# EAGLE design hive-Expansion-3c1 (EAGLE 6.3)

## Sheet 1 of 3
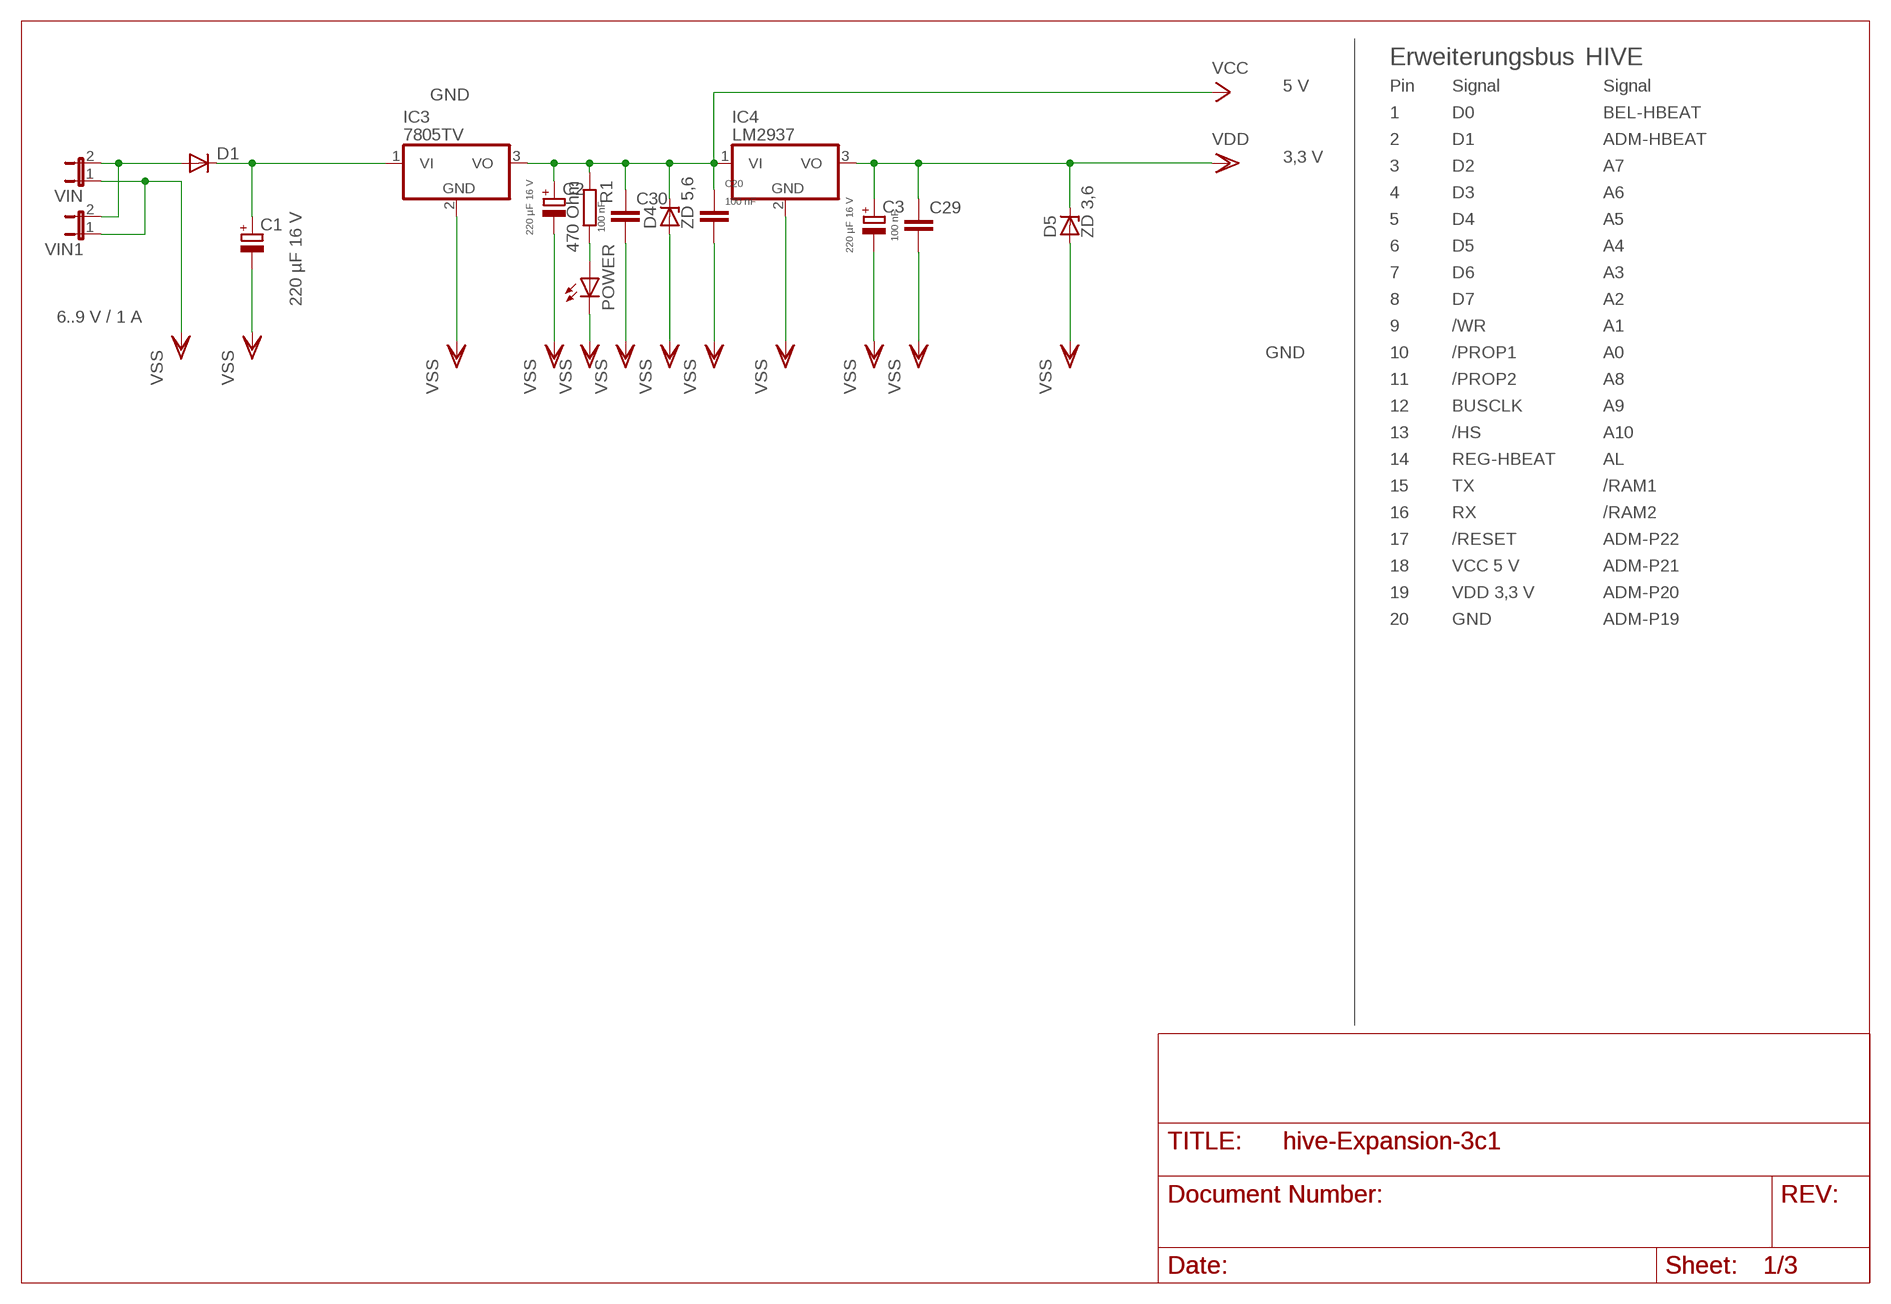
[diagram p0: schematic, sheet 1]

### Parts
C1  220 µF 16 V  CPOL-EUE3.5-10  [E3,5-10]
C2  220 µF 16 V  CPOL-EUE3.5-10  [E3,5-10]
C3  220 µF 16 V  CPOL-EUE3.5-10  [E3,5-10]
C20  100 nF  C5/2.5  [C5B2.5]
C29  100 nF  C5/2.5  [C5B2.5]
C30  100 nF  C5/2.5  [C5B2.5]
D1  DIODE-D-7.5  [D-7.5]
D4  ZD 5,6  ZENER-DIODEDO34-7  [DO34Z7]
D5  ZD 3,6  ZENER-DIODEDO34-7  [DO34Z7]
IC3  7805TV  [TO220V]
IC4  LM2937  7805TV  [TO220V]
POWER  LED5MM  [LED5MM]
R1  470 Ohm  R-EU_0204/2V  [0204V]
VIN  JP1E  [JP1]
VIN1  JP1E  [JP1]

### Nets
N$1 [Power]: D1.A VIN1.2 VIN.2
N$2 [Power]: C1.+ D1.C IC3.1(VI)
N$5: POWER.A R1.2
VCC [Power]: C2.+ C20.1 C30.1 D4.C IC3.3(VO) IC4.1(VI) R1.1 ; also sheet 3
VDD [Power]: C3.+ C29.1 D5.C IC4.3(VO) ; also sheet 2,3
VSS [Power]: C1.- C2.- C3.- C20.2 C29.2 C30.2 D4.A D5.A IC3.2(GND) IC4.2(GND) POWER.K(C) VIN1.1 VIN.1 ; also sheet 2,3

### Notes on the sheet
- Erweiterungsbus | HIVE
- 5 V | Pin | Signal | Signal
- GND
- 1 | D0 | BEL-HBEAT
- 2 | D1 | ADM-HBEAT
- 3,3 V
- 3 | D2 | A7
- 4 | D3 | A6
- 5 | D4 | A5
- 6 | D5 | A4
- 7 | D6 | A3
- 8 | D7 | A2
- 6..9 V / 1 A
- 9 | /WR | A1
- GND | 10 | /PROP1 | A0
- 11 | /PROP2 | A8
- 12 | BUSCLK | A9
- 13 | /HS | A10
- 14 | REG-HBEAT | AL
- 15 | TX | /RAM1
- 16 | RX | /RAM2
- 17 | /RESET | ADM-P22
- 18 | VCC 5 V | ADM-P21
- 19 | VDD 3,3 V | ADM-P20
- 20 | GND | ADM-P19

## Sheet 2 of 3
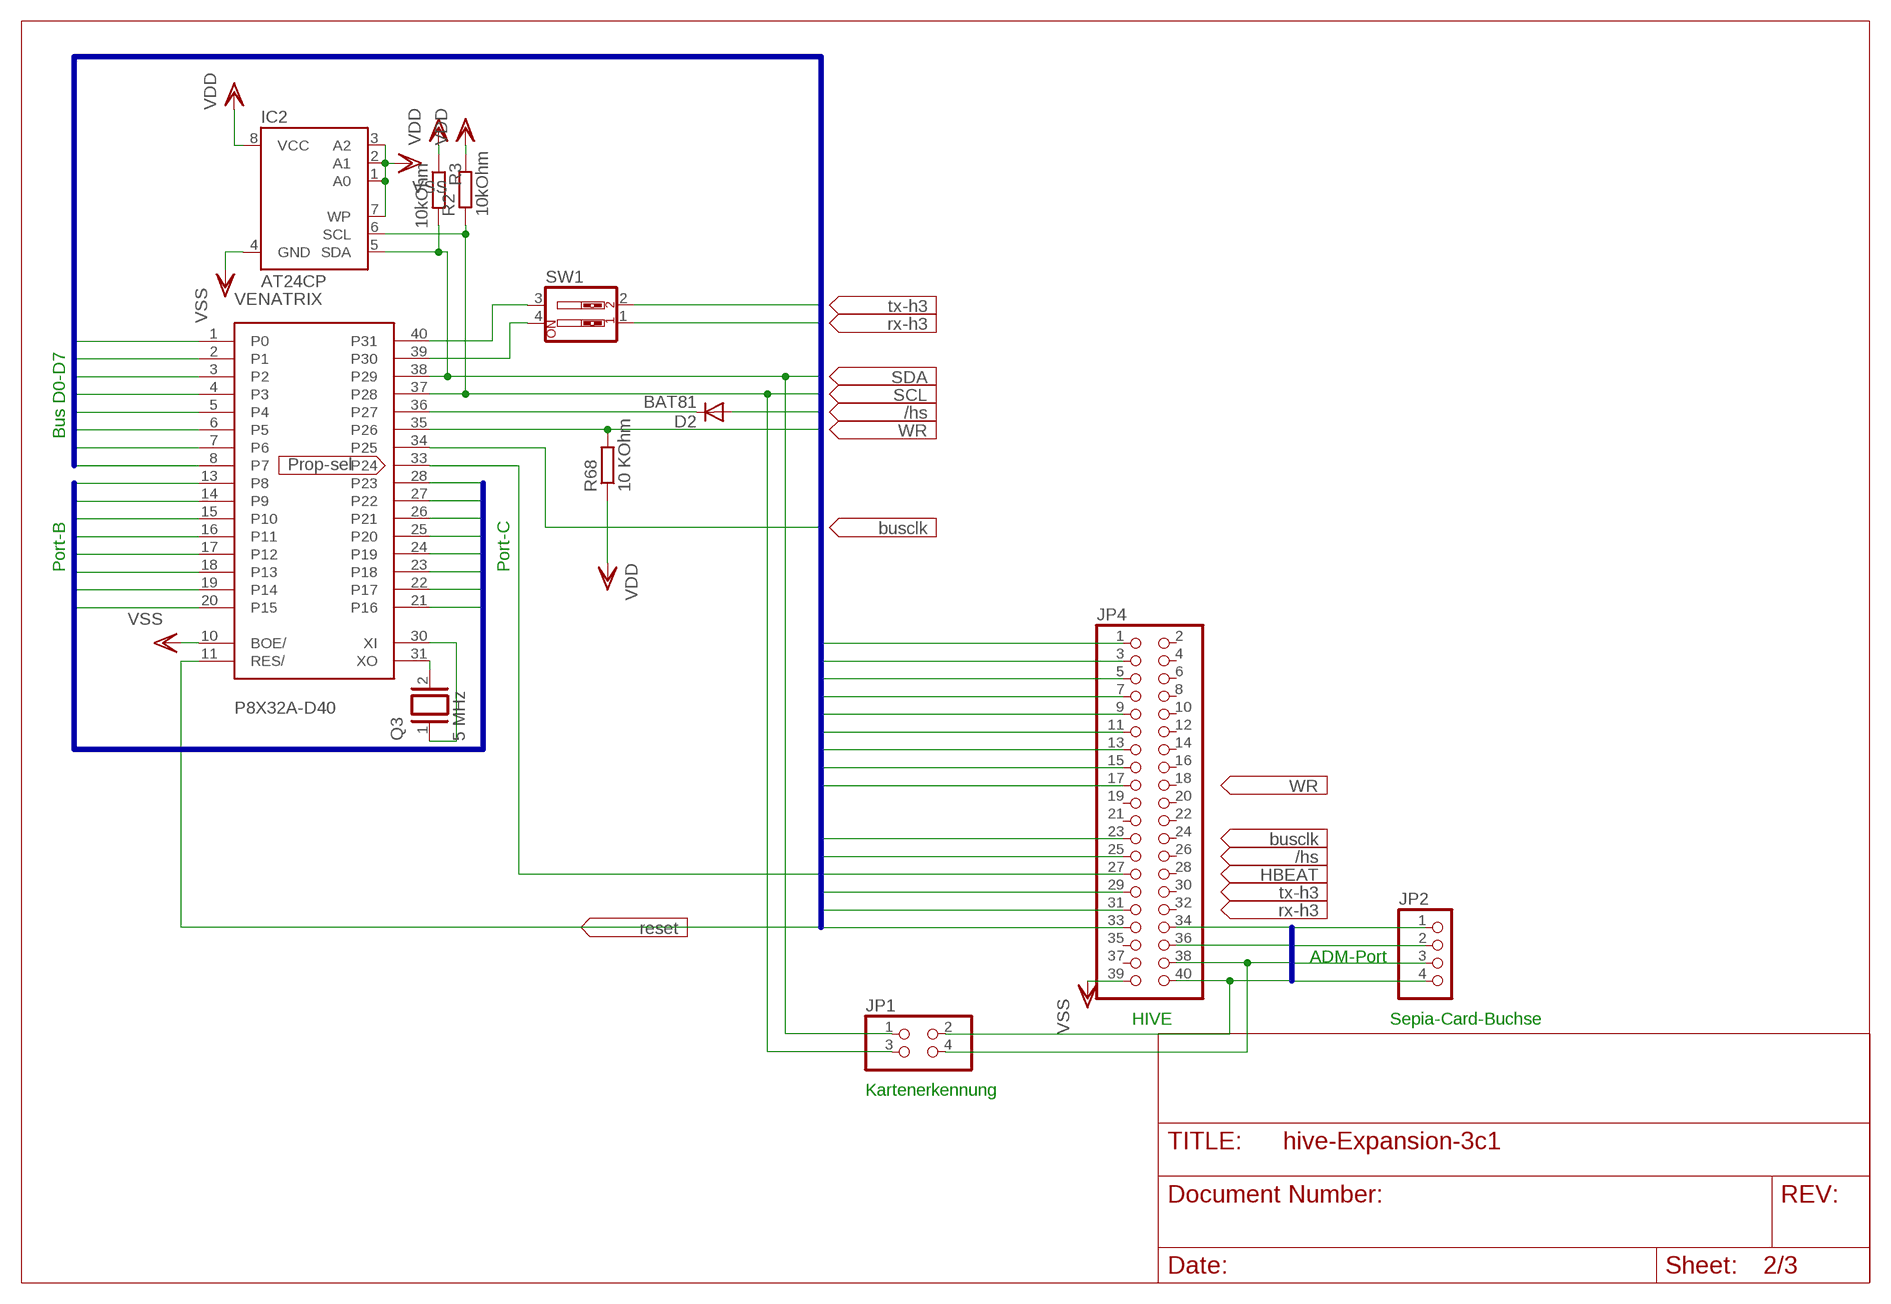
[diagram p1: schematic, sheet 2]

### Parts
D2  BAT81  [DO34-7]
IC2  AT24CP  [DIL08]
JP1  PINHD-2X2  [2X02]
JP2  PINHD-1X4  [1X04]
JP4  PINHD-2X20  [2X20]
Q3  5 MHz  XTAL/S  [QS]
R2  10kOhm  R-EU_0204/2V  [0204V]
R3  10kOhm  R-EU_0204/2V  [0204V]
R68  10 KOhm  R-EU_0204/2V  [0204V]
SW1  SW_DIP-2  [EDG-02]
VENATRIX  P8X32A-D40  [P8X32A-D40]

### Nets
EXPANSIONA1: JP4.1 VENATRIX.1(P0) ; also sheet 3
EXPANSIONA2: JP4.3 VENATRIX.2(P1) ; also sheet 3
EXPANSIONA3: JP4.5 VENATRIX.3(P2) ; also sheet 3
EXPANSIONA4: JP4.7 VENATRIX.4(P3) ; also sheet 3
EXPANSIONA5: JP4.9 VENATRIX.5(P4) ; also sheet 3
EXPANSIONA6: JP4.11 VENATRIX.6(P5) ; also sheet 3
EXPANSIONA7: JP4.13 VENATRIX.7(P6) ; also sheet 3
EXPANSIONA8: JP4.15 VENATRIX.8(P7) ; also sheet 3
EXPANSIONA9: JP4.17 R68.2 VENATRIX.35(P26) ; also sheet 3
EXPANSIONA10: IC2.5(SDA) JP1.1 R3.2 VENATRIX.38(P29) ; also sheet 3
EXPANSIONA11: IC2.6(SCL) JP1.3 R2.1 VENATRIX.37(P28) ; also sheet 3
EXPANSIONA12: JP4.23 VENATRIX.34(P25) ; also sheet 3
EXPANSIONA13: D2.A JP4.25 ; also sheet 3
EXPANSIONA14: JP4.29 SW1.1 ; also sheet 3
EXPANSIONA15: JP4.31 SW1.2 ; also sheet 3
EXPANSIONA16: JP4.33 VENATRIX.11(RES/) ; also sheet 3
EXPANSIONB1: VENATRIX.13(P8) ; also sheet 3
EXPANSIONB2: VENATRIX.14(P9) ; also sheet 3
EXPANSIONB3: VENATRIX.15(P10) ; also sheet 3
EXPANSIONB4: VENATRIX.16(P11) ; also sheet 3
EXPANSIONB5: VENATRIX.17(P12) ; also sheet 3
EXPANSIONB6: VENATRIX.18(P13) ; also sheet 3
EXPANSIONB7: VENATRIX.19(P14) ; also sheet 3
EXPANSIONB8: VENATRIX.20(P15) ; also sheet 3
EXPANSIONB9: VENATRIX.28(P23) ; also sheet 3
EXPANSIONB10: VENATRIX.27(P22) ; also sheet 3
EXPANSIONB11: VENATRIX.26(P21) ; also sheet 3
EXPANSIONB12: VENATRIX.25(P20) ; also sheet 3
EXPANSIONB13: VENATRIX.24(P19) ; also sheet 3
EXPANSIONB14: VENATRIX.23(P18) ; also sheet 3
EXPANSIONB15: VENATRIX.22(P17) ; also sheet 3
EXPANSIONB16: VENATRIX.21(P16) ; also sheet 3
EXPANSIONB17: JP2.1 JP4.34 ; also sheet 3
EXPANSIONB18: JP2.2 JP4.36 ; also sheet 3
EXPANSIONB19: JP1.4 JP2.3 JP4.38 ; also sheet 3
EXPANSIONB20: JP1.2 JP2.4 JP4.40 ; also sheet 3
N$3: D2.C VENATRIX.36(P27)
N$4: SW1.4 VENATRIX.39(P30)
N$6: SW1.3 VENATRIX.40(P31)
N$7: JP4.27 VENATRIX.33(P24)
N$65: Q3.2 VENATRIX.31(XO)
N$66: Q3.1 VENATRIX.30(XI)
VDD [Power]: IC2.8(VCC) R2.2 R3.1 R68.1 ; also sheet 1,3
VSS [Power]: IC2.1(A0) IC2.2(A1) IC2.3(A2) IC2.4(GND) IC2.7(WP) JP4.39 VENATRIX.10(BOE/) ; also sheet 1,3
Unconnected: JP4.2 JP4.4 JP4.6 JP4.8 JP4.10 JP4.12 JP4.14 JP4.16 JP4.18 JP4.19 JP4.20 JP4.21 JP4.22 JP4.24 JP4.26 JP4.28 JP4.30 JP4.32 JP4.35 JP4.37

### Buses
EXPANSIONA[1..22]
EXPANSIONB[1..22]

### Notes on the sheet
- Bus D0-D7
- Port-B | Port-C
- ADM-Port
- HIVE | Sepia-Card-Buchse
- Kartenerkennung

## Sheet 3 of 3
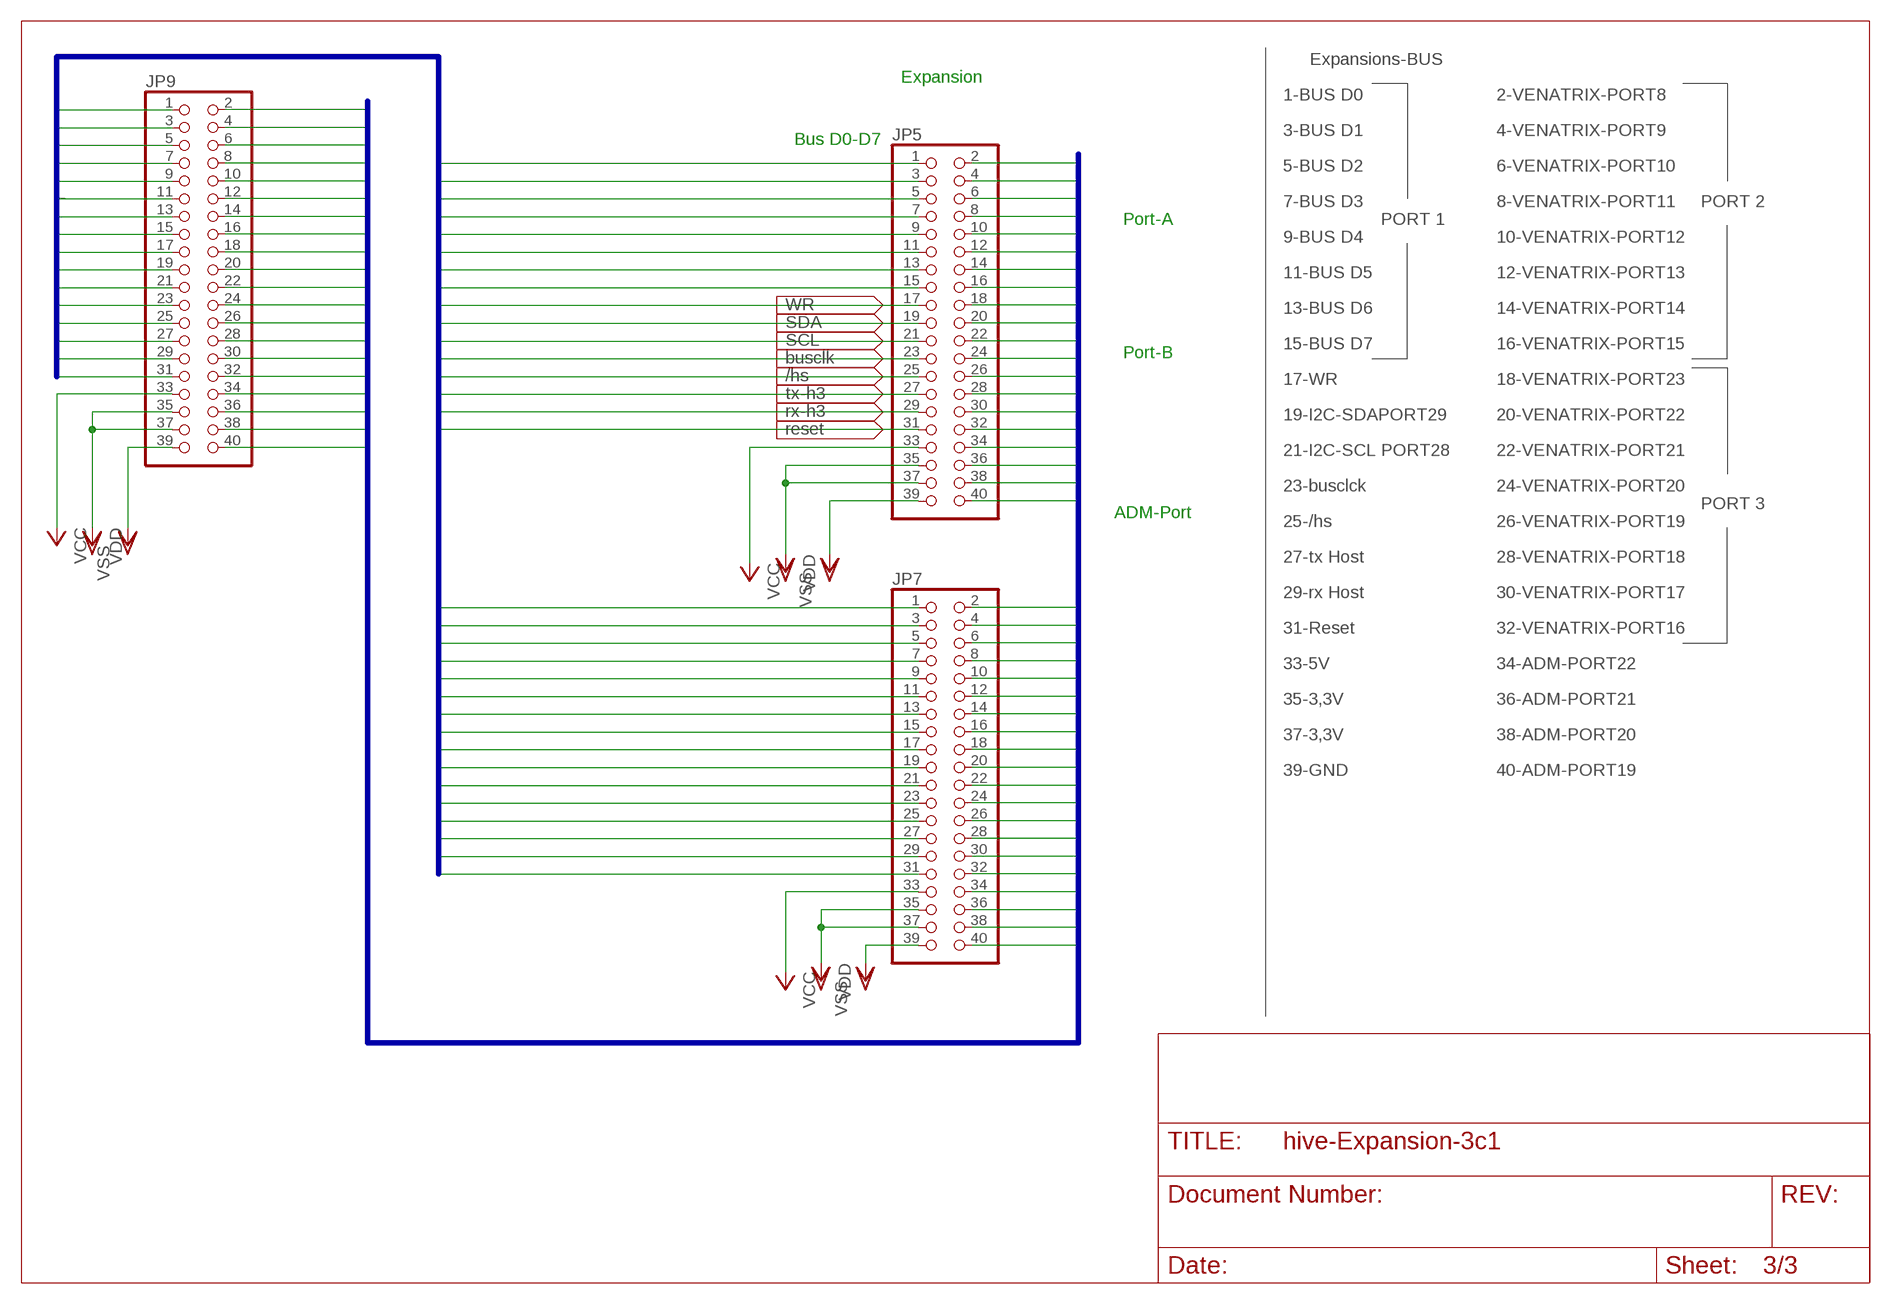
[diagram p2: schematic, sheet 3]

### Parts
JP5  PINHD-2X20  [2X20]
JP7  PINHD-2X20  [2X20]
JP9  PINHD-2X20  [2X20]

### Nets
EXPANSIONA1: JP5.1 JP7.1 JP9.1 ; also sheet 2
EXPANSIONA2: JP5.3 JP7.3 JP9.3 ; also sheet 2
EXPANSIONA3: JP5.5 JP7.5 JP9.5 ; also sheet 2
EXPANSIONA4: JP5.7 JP7.7 JP9.7 ; also sheet 2
EXPANSIONA5: JP5.9 JP7.9 JP9.9 ; also sheet 2
EXPANSIONA6: JP5.11 JP7.11 JP9.11 ; also sheet 2
EXPANSIONA7: JP5.13 JP7.13 JP9.13 ; also sheet 2
EXPANSIONA8: JP5.15 JP7.15 JP9.15 ; also sheet 2
EXPANSIONA9: JP5.17 JP7.17 JP9.17 ; also sheet 2
EXPANSIONA10: JP5.19 JP7.19 JP9.19 ; also sheet 2
EXPANSIONA11: JP5.21 JP7.21 JP9.21 ; also sheet 2
EXPANSIONA12: JP5.23 JP7.23 JP9.23 ; also sheet 2
EXPANSIONA13: JP5.25 JP7.25 JP9.25 ; also sheet 2
EXPANSIONA14: JP5.27 JP7.27 JP9.27 ; also sheet 2
EXPANSIONA15: JP5.29 JP7.29 JP9.29 ; also sheet 2
EXPANSIONA16: JP5.31 JP7.31 JP9.31 ; also sheet 2
EXPANSIONB1: JP5.2 JP7.2 JP9.2 ; also sheet 2
EXPANSIONB2: JP5.4 JP7.4 JP9.4 ; also sheet 2
EXPANSIONB3: JP5.6 JP7.6 JP9.6 ; also sheet 2
EXPANSIONB4: JP5.8 JP7.8 JP9.8 ; also sheet 2
EXPANSIONB5: JP5.10 JP7.10 JP9.10 ; also sheet 2
EXPANSIONB6: JP5.12 JP7.12 JP9.12 ; also sheet 2
EXPANSIONB7: JP5.14 JP7.14 JP9.14 ; also sheet 2
EXPANSIONB8: JP5.16 JP7.16 JP9.16 ; also sheet 2
EXPANSIONB9: JP5.18 JP7.18 JP9.18 ; also sheet 2
EXPANSIONB10: JP5.20 JP7.20 JP9.20 ; also sheet 2
EXPANSIONB11: JP5.22 JP7.22 JP9.22 ; also sheet 2
EXPANSIONB12: JP5.24 JP7.24 JP9.24 ; also sheet 2
EXPANSIONB13: JP5.26 JP7.26 JP9.26 ; also sheet 2
EXPANSIONB14: JP5.28 JP7.28 JP9.28 ; also sheet 2
EXPANSIONB15: JP5.30 JP7.30 JP9.30 ; also sheet 2
EXPANSIONB16: JP5.32 JP7.32 JP9.32 ; also sheet 2
EXPANSIONB17: JP5.34 JP7.34 JP9.34 ; also sheet 2
EXPANSIONB18: JP5.36 JP7.36 JP9.36 ; also sheet 2
EXPANSIONB19: JP5.38 JP7.38 JP9.38 ; also sheet 2
EXPANSIONB20: JP5.40 JP7.40 JP9.40 ; also sheet 2
VCC [Power]: JP5.33 JP7.33 JP9.33 ; also sheet 1
VDD [Power]: JP5.35 JP5.37 JP7.35 JP7.37 JP9.35 JP9.37 ; also sheet 1,2
VSS [Power]: JP5.39 JP7.39 JP9.39 ; also sheet 1,2

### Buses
EXPANSIONA[1..22]
EXPANSIONB[1..22]

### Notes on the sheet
- Expansions-BUS
- Expansion
- 1-BUS D0 | 2-VENATRIX-PORT8
- 3-BUS D1 | 4-VENATRIX-PORT9
- Bus D0-D7
- 5-BUS D2 | 6-VENATRIX-PORT10
- 7-BUS D3 | 8-VENATRIX-PORT11 | PORT 2
- Port-A | PORT 1
- 9-BUS D4 | 10-VENATRIX-PORT12
- 11-BUS D5 | 12-VENATRIX-PORT13
- 13-BUS D6 | 14-VENATRIX-PORT14
- 15-BUS D7 | 16-VENATRIX-PORT15
- Port-B
- 17-WR | 18-VENATRIX-PORT23
- 19-I2C-SDAPORT29 | 20-VENATRIX-PORT22
- 21-I2C-SCL PORT28 | 22-VENATRIX-PORT21
- 23-busclck | 24-VENATRIX-PORT20
- PORT 3
- ADM-Port
- 25-/hs | 26-VENATRIX-PORT19
- 27-tx Host | 28-VENATRIX-PORT18
- 29-rx Host | 30-VENATRIX-PORT17
- 31-Reset | 32-VENATRIX-PORT16
- 33-5V | 34-ADM-PORT22
- 35-3,3V | 36-ADM-PORT21
- 37-3,3V | 38-ADM-PORT20
- 39-GND | 40-ADM-PORT19

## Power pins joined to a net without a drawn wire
VDD: VENATRIX.12(VDD) VENATRIX.32(VDD)
VSS: VENATRIX.9(VSS) VENATRIX.29(VSS)

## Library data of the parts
C1-C3 = rcl:CPOL-EU: POLARIZED CAPACITOR, European symbol
C20 C29 C30 = capacitor-wima:C: CAPACITOR
D1 = diode:DIODE-: DIODE
D2 = diode:BAT81: DIODE
D4 D5 = diode:ZENER-DIODE: Z-Diode
IC2 = atmel:AT24C*: 2-wire serial EEPROM; MPN: AT24C1024BW-SH-B; OC_FARNELL: 1362646; OC_NEWARK: 03P2044
IC3 IC4 = linear:78*: Positive VOLTAGE REGULATOR Source: http://cache.national.com/ds/LM/LM78L05.pdf http://www.fairchildsemi.com/ds/LM/LM7805.pdf
JP1 = pinhead:PINHD-2X2: PIN HEADER
JP2 = pinhead:PINHD-1X4: PIN HEADER
JP4 JP5 JP7 JP9 = pinhead:PINHD-2X20: PIN HEADER
POWER = led:LED: LED
Q3 = special:XTAL/S: CRYSTAL
R1-R3 R68 = rcl:R-EU_: RESISTOR, European symbol
SW1 = special:SW_DIP-2: DIP SWITCH
VENATRIX = parallax_propeller:P8X32A-D40
VIN VIN1 = jumper:JP1E: JUMPER

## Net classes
0 default: width 0.254 mm, clearance 0.254 mm
1 Power: width 0.635 mm, drill 0.61 mm, clearance 0.381 mm
2 AudioVideo: width 0.254 mm, clearance 0.254 mm
3 Priority: width 0.279 mm, clearance 0.279 mm

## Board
Hive-Expansionsport-Platine Diese Variante soll Huckepack auf die Hive-Platine montiert werden
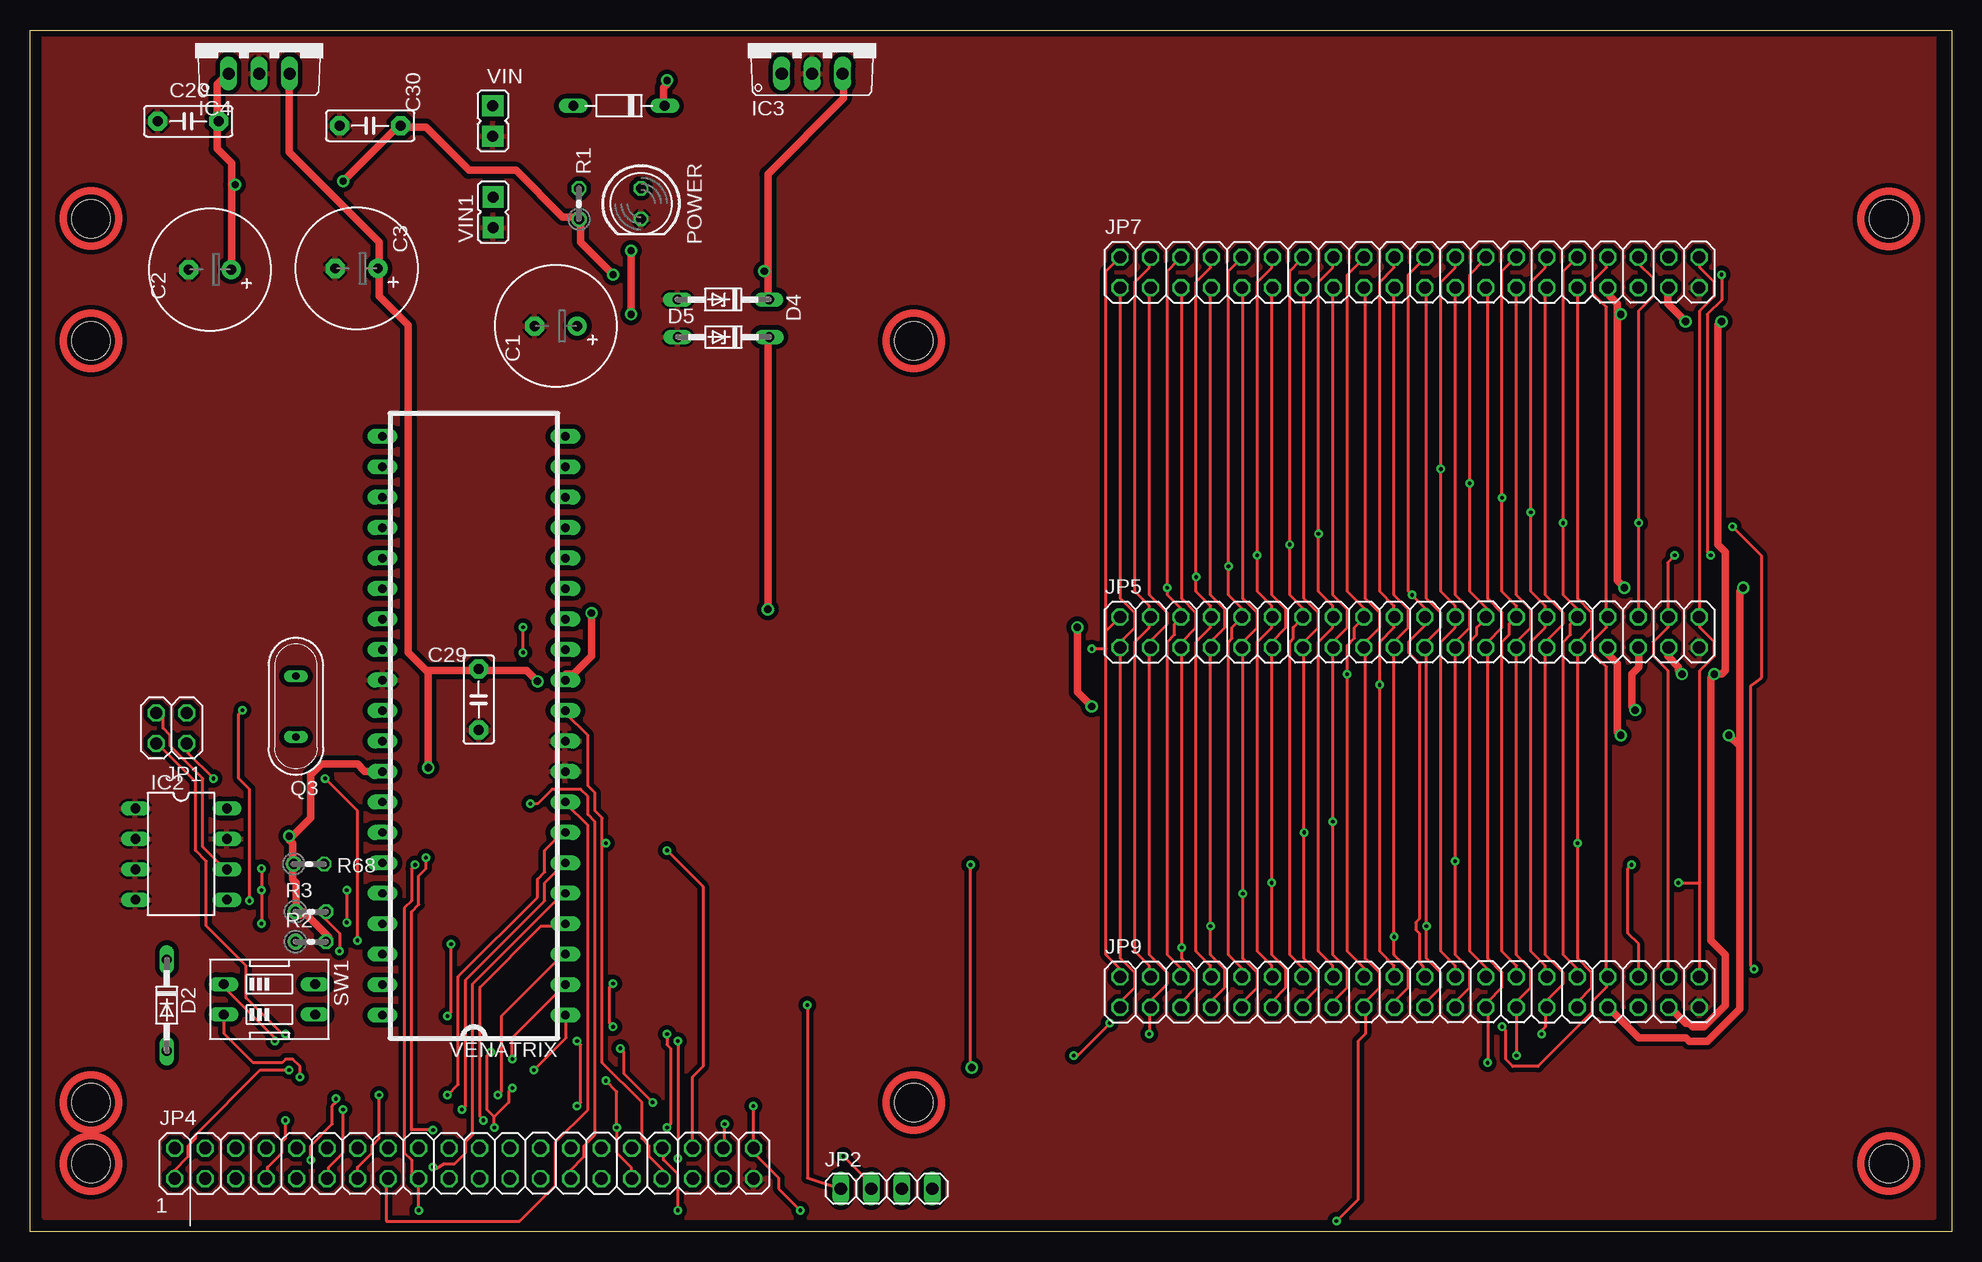
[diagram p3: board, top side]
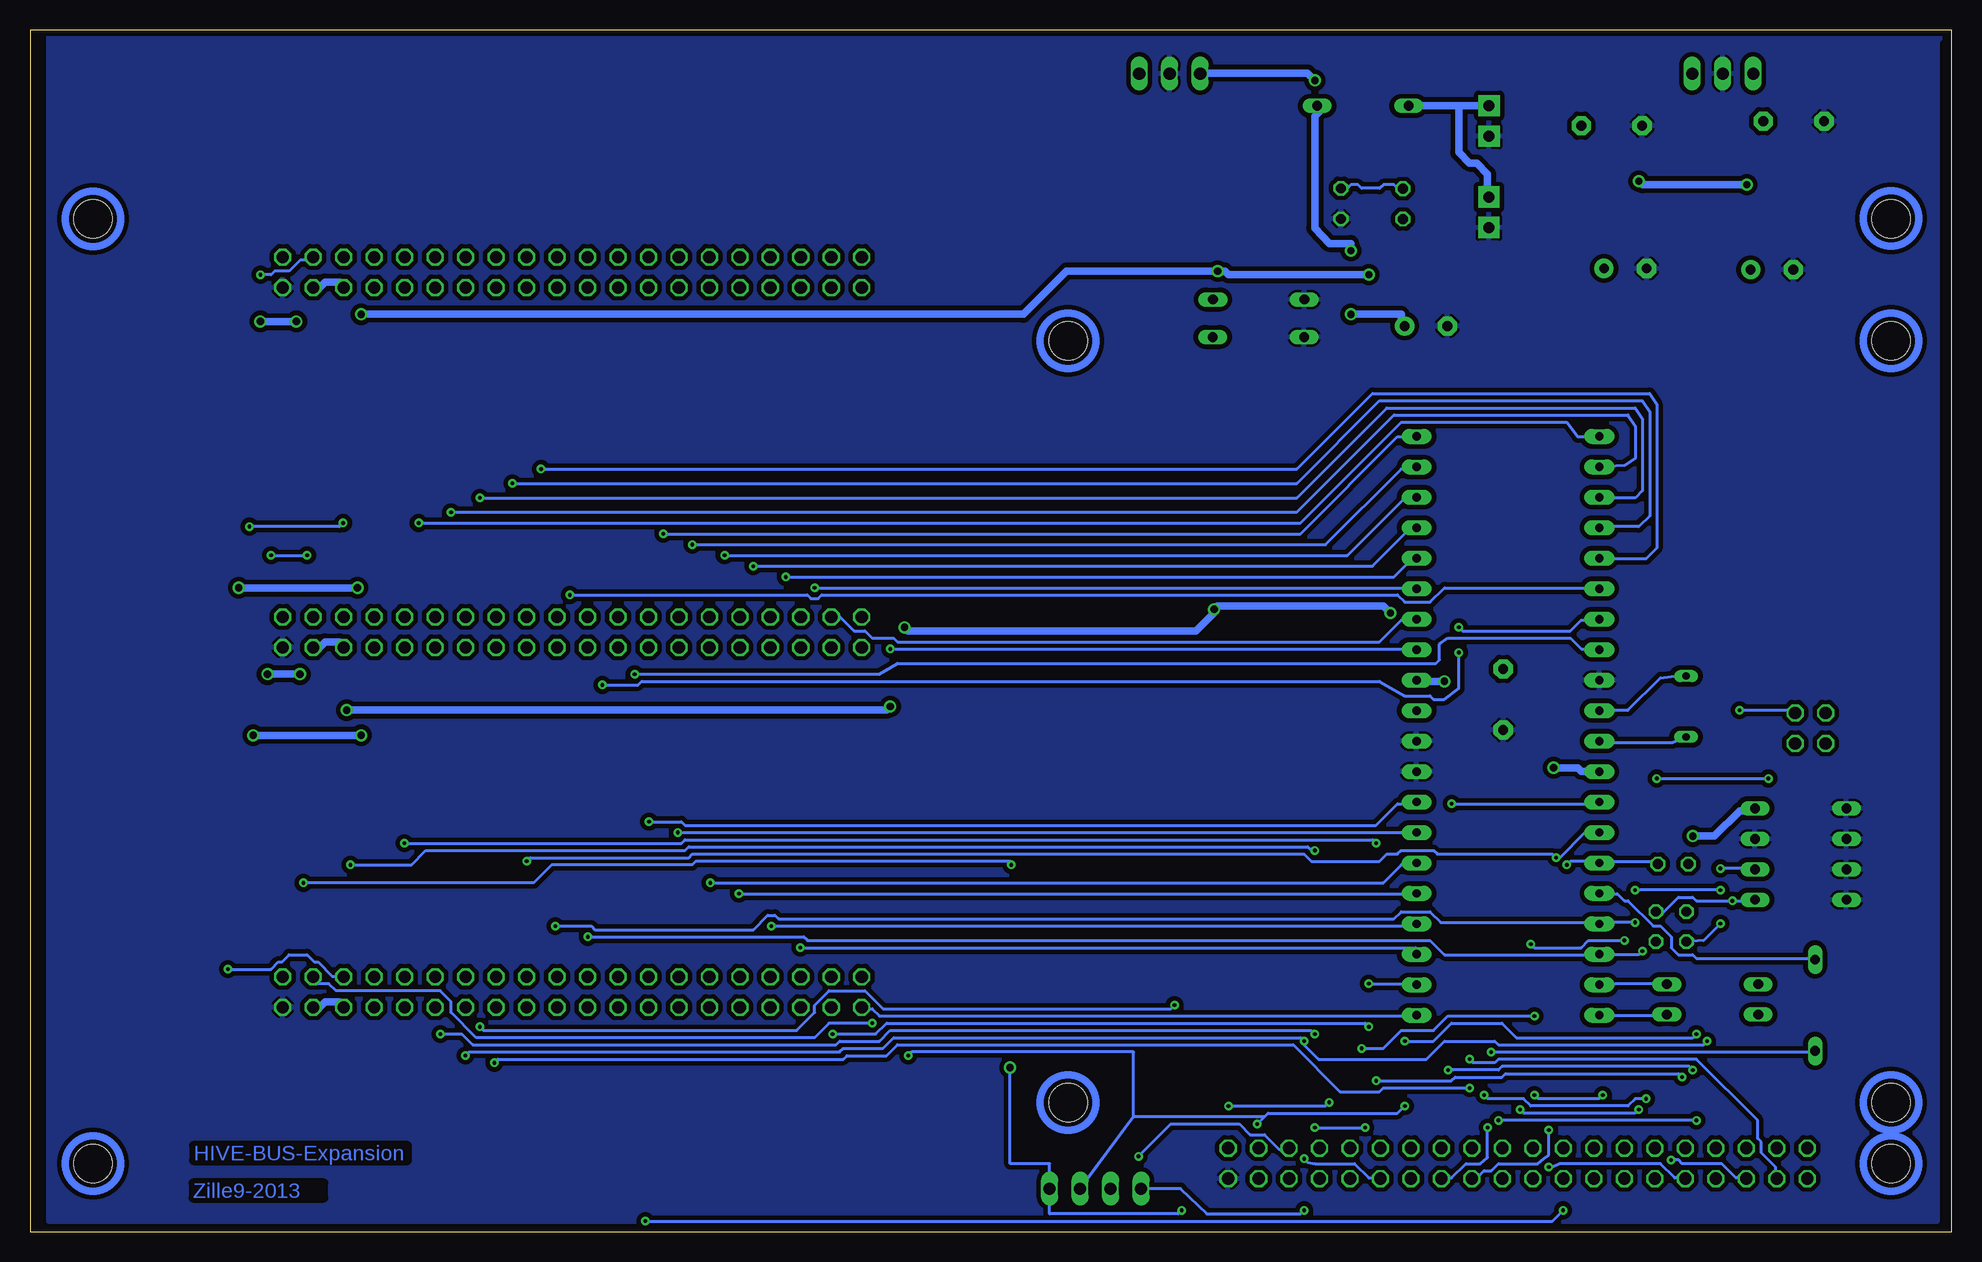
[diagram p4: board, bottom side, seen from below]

Size 160.2 x 100.2 mm. Coordinates in mm from the lower left corner, seen from the top.
Outline: 0,0 0,100.2 160.2,100.2 160.2,0 0,0
Copper layers (1*16): Top 0.035mm / dielectric 1.5mm / Bottom 0.035mm
Design rules "PCB-POOL": minimum track width 6mil, minimum drill 12mil, track to track 6mil, track to pad 6mil, pad to pad 6mil, via to via 6mil, smd to smd 6mil, copper to edge 20mil, drill to drill 8mil, minimum pad ring 8mil, minimum via ring 8mil, stop-mask expansion 3mil, vias tented up to drill 24mil, thermal gap 8mil
Holes 3.2 mm at 73.66,74.3 5.08,74.3 5.08,10.79 73.66,10.79 154.94,84.46 154.94,5.71 5.08,84.45 5.08,5.71

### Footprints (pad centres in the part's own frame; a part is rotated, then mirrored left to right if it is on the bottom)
E3,5-10 = drill 0.813 pad 1.6: + -1.778,0 | drill 0.813 pad 1.6 octagon: - 1.778,0
C5B2.5 = drill 0.813 pad 1.6 octagon: 1 -2.54,0; 2 2.54,0
D-7.5 = drill 0.813 long: A 3.81,0; C -3.81,0
DO34-7 = drill 0.813 long: A 3.81,0; C -3.81,0
DO34Z7 = drill 0.813 long: A 3.81,0; C -3.81,0
DIL08 = drill 0.813 long: 1 -3.81,-3.81; 2 -1.27,-3.81; 3 1.27,-3.81; 4 3.81,-3.81; 5 3.81,3.81; 6 1.27,3.81; 7 -1.27,3.81; 8 -3.81,3.81
TO220V = drill 1.016 long: 1 -2.54,-2.54; 2 0,-2.54; 3 2.54,-2.54
2X02 = drill 1.016 octagon: 1 -1.27,-1.27; 2 -1.27,1.27; 3 1.27,-1.27; 4 1.27,1.27
1X04 = drill 1.016 long: 1 -3.81,0; 2 -1.27,0; 3 1.27,0; 4 3.81,0
2X20 = drill 1.016 octagon: 1 -24.13,-1.27; 2 -24.13,1.27; 3 -21.59,-1.27; 4 -21.59,1.27; 5 -19.05,-1.27; 6 -19.05,1.27; 7 -16.51,-1.27; 8 -16.51,1.27; 9 -13.97,-1.27; 10 -13.97,1.27; 11 -11.43,-1.27; 12 -11.43,1.27; 13 -8.89,-1.27; 14 -8.89,1.27; 15 -6.35,-1.27; 16 -6.35,1.27; 17 -3.81,-1.27; 18 -3.81,1.27; 19 -1.27,-1.27; 20 -1.27,1.27; 21 1.27,-1.27; 22 1.27,1.27; 23 3.81,-1.27; 24 3.81,1.27; 25 6.35,-1.27; 26 6.35,1.27; 27 8.89,-1.27; 28 8.89,1.27; 29 11.43,-1.27; 30 11.43,1.27; 31 13.97,-1.27; 32 13.97,1.27; 33 16.51,-1.27; 34 16.51,1.27; 35 19.05,-1.27; 36 19.05,1.27; 37 21.59,-1.27; 38 21.59,1.27; 39 24.13,-1.27; 40 24.13,1.27
LED5MM = drill 0.813 octagon: A -1.27,0; K 1.27,0
QS = drill 0.61 long: 1 -2.54,0; 2 2.54,0
0204V = drill 0.813 octagon: 1 -1.27,0; 2 1.27,0
EDG-02 = drill 0.813 long: 1 -1.27,-3.81; 2 1.27,-3.81; 3 1.27,3.81; 4 -1.27,3.81
P8X32A-D40 = drill 0.7 pad 1.27 long: 1 -7.62,23.495; 2 -7.62,20.955; 3 -7.62,18.415; 4 -7.62,15.875; 5 -7.62,13.335; 6 -7.62,10.795; 7 -7.62,8.255; 8 -7.62,5.715; 9 -7.62,3.175; 10 -7.62,0.635; 11 -7.62,-1.905; 12 -7.62,-4.445; 13 -7.62,-6.985; 14 -7.62,-9.525; 15 -7.62,-12.065; 16 -7.62,-14.605; 17 -7.62,-17.145; 18 -7.62,-19.685; 19 -7.62,-22.225; 20 -7.62,-24.765; 21 7.62,-24.765; 22 7.62,-22.225; 23 7.62,-19.685; 24 7.62,-17.145; 25 7.62,-14.605; 26 7.62,-12.065; 27 7.62,-9.525; 28 7.62,-6.985; 29 7.62,-4.445; 30 7.62,-1.905; 31 7.62,0.635; 32 7.62,3.175; 33 7.62,5.715; 34 7.62,8.255; 35 7.62,10.795; 36 7.62,13.335; 37 7.62,15.875; 38 7.62,18.415; 39 7.62,20.955; 40 7.62,23.495
JP1 = drill 0.914 pad 1.778 square: 1 0,-1.27; 2 0,1.27

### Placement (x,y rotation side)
C1  43.84,75.52 180 top
C2  15,80.22 180 top
C3  27.22,80.32 180 top
C20  13.19,92.59 180 top
C29  37.4,44.39 270 top
C30  28.36,92.22 180 top
D1  49.09,93.89 180 top
D2  11.4,18.9 270 top
D4  57.79,77.73 180 top
D5  57.81,74.6 180 top
IC2  12.6,31.5 270 top
IC3  65.2,99.1 0 top
IC4  19.1,99.1 0 top
JP1  11.8,42 180 top
JP2  71.4,3.6 0 top
JP4  36.2,5.71 0 top
JP5  115,50 0 top
JP7  115,80 0 top
JP9  115,20 0 top
POWER  50.93,85.73 270 top
Q3  22.16,43.8 270 top
R1  45.76,85.71 90 top
R2  23.4,24.2 0 top
R3  23.4,26.7 0 top
R68  23.24,30.67 0 top
SW1  19.95,19.39 270 top
VENATRIX  37,41.56 180 top
VIN  38.58,92.62 0 top
VIN1  38.6,85 0 top

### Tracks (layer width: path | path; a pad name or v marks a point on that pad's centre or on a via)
EXPANSIONA1  (via drill 0.3)
  Top 0.254: v42,13.5 44.7,16.2 44.7,18 VENATRIX.1 | v21.6,13.5 19.2,13.5 13.8,8.1 13.8,7.8 13.2,7.2 13.2,6.3 12,5.1 12,4.5 JP4.1 | JP9.1 90.9,18.9 90.9,19.2 92.1,20.4 92.1,21.6 90.9,22.8 90.9,48.6 JP5.1 90.9,48.9 90.9,49.2 92.1,50.4 92.1,51.6 90.9,52.8 90.9,78.6 JP7.1
  Bottom 0.254: v42,13.5 37.8,13.5 37.5,13.8 21.9,13.8 v21.6,13.5 | VENATRIX.1 44.7,18 89.4,18 90,18.6 90.6,18.6 JP9.1
EXPANSIONA2  (via drill 0.3)
  Top 0.254: v40.2,14.4 40.2,16.2 44.4,20.4 VENATRIX.2 | JP7.3 93.3,78.6 93.3,53.1 94.8,51.6 94.8,50.7 93.3,49.2 93.3,48.9 JP5.3 93.3,48.6 93.3,23.1 94.8,21.6 94.8,20.7 93.3,19.2 93.3,18.9 JP9.3 93.3,18.6 v93.3,16.5 | v48.6,20.7 48.3,20.4 48.3,17.4 v48.6,17.1
  Bottom 0.254: v40.2,14.4 39.9,14.1 38.1,14.1 37.8,14.4 21.3,14.4 16.2,9.3 16.2,7.8 15.9,7.5 15.9,6.6 14.7,5.4 14.7,4.5 JP4.3 | v48.6,20.7 44.7,20.7 VENATRIX.2 | v48.6,17.1 48.9,17.4 88.8,17.4 89.7,16.5 v93.3,16.5
EXPANSIONA3  (via drill 0.3)
  Top 0.254: v39,11.4 39.3,11.7 39.3,18 44.4,23.1 VENATRIX.3 | v25.5,11.1 25.5,10.8 25.2,10.5 25.2,9 23.4,7.2 v23.4,6 | JP9.5 96,18.9 96,19.2 97.2,20.4 97.2,21.6 96,22.8 v96,23.7 96,48.6 JP5.5 96,48.9 96,49.2 97.2,50.4 97.2,51.6 96,52.8 96,78.6 JP7.5
  Bottom 0.254: v39,11.4 38.7,11.1 35.7,11.1 35.1,10.5 27,10.5 26.4,11.1 v25.5,11.1 | v23.4,6 22.8,6 22.5,5.7 19.2,5.7 18,4.5 17.4,4.5 JP4.5 | v96,23.7 44.7,23.7 VENATRIX.3
EXPANSIONA4  (via drill 0.3)
  Top 0.254: v37.8,9.3 37.5,9.6 37.5,20.4 42.6,25.5 44.4,25.5 VENATRIX.4 | v21.3,9.3 21.3,7.8 21,7.5 21,6.6 19.8,5.4 19.8,4.5 JP4.7 | JP9.7 98.4,18.9 98.4,19.2 99.6,20.4 99.6,21.9 98.4,23.1 v98.4,25.5 98.4,48.6 JP5.7 98.4,48.9 98.4,49.2 99.6,50.4 99.6,51.9 98.4,53.1 98.4,78.6 JP7.7
  Bottom 0.254: v21.3,9.3 v37.8,9.3 | v98.4,25.5 44.7,25.5 VENATRIX.4
EXPANSIONA5  (via drill 0.3)
  Top 0.254: v33.6,5.4 33.9,5.3 34.5,5.7 35.4,5.7 36.3,6.6 36.3,7.5 36.9,8.1 36.9,20.7 44.4,28.2 VENATRIX.5 | JP9.9 101.1,18.9 101.1,19.2 102.3,20.4 102.3,21.6 101.1,22.8 v101.1,28.2 101.1,48.6 JP5.9 101.1,48.9 101.1,49.2 102.3,50.4 102.3,51.6 101.1,52.8 101.1,78.6 JP7.9
  Bottom 0.254: v33.6,5.4 33.3,5.4 32.7,5.7 24.3,5.7 23.1,4.5 22.5,4.5 JP4.9 | v101.1,28.2 44.7,28.2 VENATRIX.5
EXPANSIONA6  (via drill 0.3)
  Top 0.254: v36,10.2 36.3,10.5 36.3,21 42.9,27.6 42.9,29.1 44.4,30.6 VENATRIX.6 | v26.1,10.2 26.1,6.6 24.9,5.4 24.9,4.5 JP4.11 | JP9.11 103.5,18.9 103.5,19.2 104.7,20.4 104.7,21.9 103.5,23.1 v103.5,29.1 103.5,48.6 JP5.11 103.5,48.9 103.5,49.2 104.7,50.4 104.7,51.9 103.5,53.1 103.5,78.6 JP7.11
  Bottom 0.254: v36,10.2 35.7,9.9 26.4,9.9 v26.1,10.2 | v103.5,29.1 47.4,29.1 45.9,30.6 44.7,30.6 VENATRIX.6
EXPANSIONA7  (via drill 0.3)
  Top 0.254: v34.8,11.4 35.7,12.3 35.7,21.3 42.3,27.9 42.3,29.4 42.9,30 42.9,31.8 44.4,33.3 VENATRIX.7 | v29.1,11.4 29.1,7.8 28.5,7.2 28.5,6.6 27.3,5.4 27.3,4.5 JP4.13 | JP9.13 106.2,18.9 106.2,19.2 107.4,20.4 107.4,21.6 106.2,22.8 v106.2,33.3 106.2,48.6 JP5.13 106.2,48.9 106.2,49.2 107.4,50.4 107.4,51.6 106.2,52.8 106.2,78.6 JP7.13
  Bottom 0.254: v34.8,11.4 34.5,11.1 29.4,11.1 v29.1,11.4 | v106.2,33.3 44.7,33.3 VENATRIX.7
EXPANSIONA8  (via drill 0.3)
  Top 0.254: VENATRIX.8 44.7,35.7 46.5,33.9 46.5,10.2 43.8,7.5 43.8,3.9 40.8,0.9 29.7,0.9 29.7,4.2 JP4.15 | JP9.15 108.6,18.9 108.6,19.2 109.8,20.4 109.8,21.9 108.6,23.1 v108.6,34.2 108.6,48.6 JP5.15 108.6,48.9 108.6,49.2 109.8,50.4 109.8,51.9 108.6,53.1 108.6,78.6 JP7.15
  Bottom 0.254: v108.6,34.2 105.9,34.2 105.6,33.9 48,33.9 46.2,35.7 44.7,35.7 VENATRIX.8
EXPANSIONA9  (via drill 0.3)
  Top 0.254: v32.1,30.6 31.8,30.3 31.8,27.6 31.2,27 31.2,6.6 31.8,6 31.8,4.8 32.1,4.5 JP4.17 32.4,4.2 v32.4,1.8 | JP7.17 111.3,78.6 111.3,52.8 112.5,51.6 112.5,50.4 111.3,49.2 111.3,48.9 JP5.17 111.3,48.6 111.3,22.8 112.5,21.6 112.5,20.4 111.3,19.2 111.3,18.9 JP9.17 111.3,18.6 111.3,16.5 110.7,15.9 110.7,2.7 v108.9,0.9
  Bottom 0.254: R68.2 24.6,30.9 29.1,30.9 VENATRIX.35 29.4,30.9 31.8,30.9 v32.1,30.6 | v32.4,1.8 33.3,0.9 v108.9,0.9
EXPANSIONA10  (via drill 0.3)
  Top 0.254: JP9.19 113.7,18.9 113.7,19.2 114.9,20.4 114.9,21.9 113.7,23.1 v113.7,24.6 113.7,48.6 JP5.19 113.7,48.9 113.7,49.2 114.9,50.4 114.9,51.9 113.7,53.1 113.7,78.6 JP7.19 | v25.8,23.4 25.8,24.9 24.6,26.1 24.6,26.7 R3.2 | v17.7,43.5 17.4,43.2 17.4,37.8 18.3,36.9 v18.3,27.6
  Bottom 0.254: R3.2 24,26.7 22.8,27.9 21.6,27.9 21.3,27.6 v18.3,27.6 16.5,27.6 IC2.5 | v25.8,23.4 26.1,23.1 29.1,23.1 VENATRIX.38 29.4,23.1 42.3,23.1 43.5,24.3 95.4,24.3 95.7,24.6 v113.7,24.6 | v17.7,43.5 13.2,43.5 JP1.1
EXPANSIONA11  (via drill 0.3)
  Top 0.254: JP9.21 116.4,18.9 116.4,19.2 117.6,20.4 117.6,21.6 116.4,22.8 v116.4,25.5 116.4,48.6 JP5.21 116.4,48.9 116.4,49.2 117.6,50.4 117.6,51.6 116.4,52.8 116.4,78.6 JP7.21 | v19.3,30.3 v19.3,28.5 v19.3,25.7 | v26.4,28.5 v26.4,25.8 | JP1.3 10.8,43.2 11.1,42.9 11.1,42 11.7,41.4 11.7,40.5 14.4,37.8 14.4,32.1 16.2,30.3 IC2.6
  Bottom 0.254: R2.1 20.7,24.3 v19.3,25.7 | v19.3,30.3 16.5,30.3 IC2.6 | v26.4,25.8 29.1,25.8 VENATRIX.37 29.4,25.8 42.6,25.8 43.5,26.7 45.9,26.7 46.5,26.1 97.8,26.1 98.1,26.4 98.7,26.4 99.9,25.2 113.1,25.2 113.4,25.5 v116.4,25.5 | v19.3,28.5 v26.4,28.5
EXPANSIONA12  (via drill 0.3)
  Top 0.254: v33,31.2 33,30.3 32.4,29.7 32.4,27.3 31.8,26.7 31.8,8.5 v33.6,8.5 | JP9.23 118.8,18.9 118.8,19.2 120,20.4 120,21.9 118.8,23.1 v118.8,30.9 118.8,48.6 JP5.23 118.8,48.9 118.8,49.2 120,50.4 120,51.9 118.8,53.1 118.8,78.6 JP7.23
  Bottom 0.254: v33.6,8.5 33.6,6.4 34,6.1 34.5,5.7 37.8,5.7 38.4,5.1 39,5.1 39.6,4.5 39.9,4.5 JP4.23 | VENATRIX.34 29.4,33.3 30.6,33.3 32.7,31.2 v33,31.2 33.3,31.5 42.9,31.5 43.2,31.8 45.9,31.8 46.2,31.5 47.1,31.5 47.7,30.9 53.4,30.9 54,31.5 105,31.5 105.3,31.2 118.5,31.2 v118.8,30.9
EXPANSIONA13  (via drill 0.3)
  Top 0.254: v38.4,15 38.1,14.7 38.1,10.2 38.7,9.6 | v38.7,8.7 38.7,9.6 | JP7.25 121.5,78.6 121.5,52.8 122.7,51.6 122.7,50.4 121.5,49.2 121.5,48.9 JP5.25 121.5,48.6 121.5,22.8 122.7,21.6 122.7,20.4 121.5,19.2 121.5,18.9 JP9.25 121.5,18.6 v121.5,14.1 | 38.7,9.6 39.9,10.8 39.9,11.7 v40.2,12
  Bottom 0.254: v38.4,15 11.4,15 D2.A | v38.7,8.7 38.7,6.2 39.3,5.7 40.5,5.7 41.7,4.5 42.3,4.5 JP4.25 | v40.2,12 47.4,12 47.7,11.7 51,11.7 54.9,15.6 87.9,15.6 88.8,14.7 92.1,14.7 92.4,14.4 121.2,14.4 v121.5,14.1
EXPANSIONA14  (via drill 0.3)
  Top 0.254: JP7.27 123.9,78.6 123.9,53.1 125.1,51.9 125.1,50.4 123.9,49.2 123.9,48.9 JP5.27 123.9,48.6 123.9,23.1 125.1,21.9 125.1,20.4 123.9,19.2 123.9,18.9 JP9.27 123.9,18.6 v123.9,14.7 | v54,15.9 v54,6.1 | v20.4,15.9 20.4,16.2 16.2,20.4 SW1.1
  Bottom 0.254: v54,6.1 53.7,5.8 53.1,5.7 49.8,5.7 48.6,4.5 47.7,4.5 JP4.29 | v123.9,14.7 123.6,15 92.7,15 92.4,15.3 89.1,15.3 88.2,16.2 54.3,16.2 v54,15.9 54,15.6 52.8,14.4 43.8,14.4 42.3,15.9 38.1,15.9 37.8,15.6 20.7,15.6 v20.4,15.9
EXPANSIONA15  (via drill 0.3)
  Top 0.254: JP7.29 126.3,78.6 126.3,53.1 127.8,51.6 127.8,50.7 126.3,49.2 126.3,48.9 JP5.29 126.3,48.6 126.3,23.1 127.8,21.6 127.8,20.7 126.3,19.2 126.3,18.9 JP9.29 126.3,18.6 126.3,17.1 126,16.8 v126,16.5 | v53.1,8.7 53.4,9 53.4,15.3 53.1,15.6 v53.1,16.5 | JP4.31 50.1,4.5 50.1,5.4 48.9,6.6 v48.9,8.7 48.9,11.7 v48,12.6 | v22.5,12.9 22.5,13.8 21.9,14.4 21.3,14.4 21,14.1 18.6,14.1 16.2,16.5 16.2,18 SW1.2
  Bottom 0.254: v53.1,8.7 v48.9,8.7 | v53.1,16.5 53.4,16.8 88.5,16.8 89.4,15.9 92.7,15.9 93,15.6 123.3,15.6 124.2,16.5 v126,16.5 | v22.5,12.9 22.8,13.2 37.2,13.2 37.5,12.9 41.4,12.9 41.7,12.6 v48,12.6
EXPANSIONA16  (via drill 0.3)
  Top 0.254: 47.7,32.4 47.7,14.1 51,10.8 51,7.8 51.6,7.2 51.6,6.3 52.8,5.1 52.8,4.5 JP4.33 | 47.7,32.4 47.7,34.5 47.1,35.1 47.1,36.6 46.5,37.2 46.5,41.4 44.7,43.2 VENATRIX.11 | JP9.31 129,18.9 129,19.2 130.2,20.4 130.2,21.6 129,22.8 v129,32.4 129,48.6 JP5.31 129,48.9 129,49.2 130.2,50.4 130.2,51.6 129,52.8 129,78.6 JP7.31 | v48,32.4 47.7,32.4
  Bottom 0.254: v48,32.4 48.3,32.7 105.6,32.7 105.9,32.4 v129,32.4
EXPANSIONB1  (via drill 0.3)
  Top 0.254: 89.7,50.1 JP5.2 | 89.7,48.6 89.7,23.1 90.9,21.9 90.9,21.3 JP9.2 | 89.7,48.6 89.7,50.1 | JP7.2 89.7,80.1 89.7,50.1 | 89.7,48.6 v88.5,48.6
  Bottom 0.254: v88.5,48.6 44.7,48.6 VENATRIX.13
EXPANSIONB2
  Top 0.254: JP9.4 93.3,21.3 93.3,22.2 92.1,23.4 92.1,49.2 93.3,50.4 93.3,51 JP5.4 93.3,51.3 93.3,52.2 92.1,53.4 92.1,79.2 93.3,80.4 93.3,81 JP7.4
  Bottom 0.254: VENATRIX.14 44.7,51 45.9,51 47.7,49.2 87.9,49.2 88.2,49.5 90,49.5 90.6,50.1 91.5,50.1 92.7,51.3 93.3,51.3 JP5.4
EXPANSIONB3  (via drill 0.3)
  Top 0.254: JP9.6 96,21.3 96,21.9 94.8,23.1 94.8,49.2 95.4,49.8 95.4,50.7 95.7,51 JP5.6 96,51.3 96,51.9 94.8,53.1 v94.8,53.7 94.8,80.1 95.7,81 JP7.6
  Bottom 0.254: v94.8,53.7 45,53.7 VENATRIX.15
EXPANSIONB4  (via drill 0.3)
  Top 0.254: JP9.8 98.4,21.3 98.4,22.2 97.2,23.4 97.2,49.2 98.4,50.4 98.4,51 JP5.8 98.4,51.3 98.4,52.2 97.2,53.4 v97.2,54.6 97.2,79.2 98.4,80.4 98.4,81 JP7.8
  Bottom 0.254: v97.2,54.6 46.5,54.6 45,56.1 VENATRIX.16
EXPANSIONB5  (via drill 0.3)
  Top 0.254: JP9.10 101.1,21.3 101.1,21.9 99.9,23.1 99.9,49.2 100.2,49.5 100.2,50.4 100.8,51 JP5.10 101.1,51.3 101.1,51.9 99.9,53.1 v99.9,55.5 99.9,80.1 100.8,81 JP7.10
  Bottom 0.254: v99.9,55.5 48.3,55.5 45.3,58.5 VENATRIX.17
EXPANSIONB6  (via drill 0.3)
  Top 0.254: JP9.12 103.5,21.3 103.5,22.2 102.3,23.4 102.3,49.2 103.5,50.4 103.5,51 JP5.12 103.5,51.3 103.5,52.2 102.3,53.4 v102.3,56.4 102.3,79.2 103.5,80.4 103.5,81 JP7.12
  Bottom 0.254: v102.3,56.4 50.4,56.4 45.6,61.2 VENATRIX.18
EXPANSIONB7  (via drill 0.3)
  Top 0.254: JP9.14 106.2,21.3 106.2,21.9 105,23.1 105,49.2 105.3,49.5 105.3,50.4 105.9,51 JP5.14 106.2,51.3 106.2,51.9 105,53.1 v105,57.3 105,80.1 105.9,81 JP7.14
  Bottom 0.254: v105,57.3 52.2,57.3 45.9,63.6 VENATRIX.19
EXPANSIONB8  (via drill 0.3)
  Top 0.254: JP9.16 108.6,21.3 108.6,22.2 107.4,23.4 107.4,49.2 108.6,50.4 108.6,51 JP5.16 108.6,51.3 108.6,52.2 107.4,53.4 v107.4,58.2 107.4,79.2 108.6,80.4 108.6,81 JP7.16
  Bottom 0.254: v107.4,58.2 54.3,58.2 46.2,66.3 VENATRIX.20
EXPANSIONB9  (via drill 0.3)
  Top 0.254: JP9.18 111.3,21.3 111.3,21.9 109.8,23.4 v109.8,46.5 109.8,48.9 110.4,49.5 110.4,50.4 111,51 JP5.18 111.3,51.3 111.3,51.9 109.8,53.4 109.8,79.8 111,81 JP7.18
  Bottom 0.254: v109.8,46.5 89.4,46.5 87.9,47.4 43,47.4 42.7,47.7 42.7,49 42,49.5 31.8,49.5 30.9,48.6 29.4,48.6 VENATRIX.28
EXPANSIONB10  (via drill 0.3)
  Top 0.254: JP9.20 113.7,21.3 113.7,22.2 112.5,23.4 v112.5,45.6 112.5,49.2 113.7,50.4 113.7,51 JP5.20 113.7,51.3 113.7,52.2 112.5,53.4 112.5,79.2 113.7,80.4 113.7,81 JP7.20 | v41.1,48.3 v41.1,50.4
  Bottom 0.254: v41.1,50.4 40.8,50.1 31.8,50.1 30.9,51 29.4,51 VENATRIX.27 | v41.1,48.3 41.1,45.3 42.3,44.4 43.2,44.4 43.5,44.7 45.6,44.7 47.7,45.9 109.2,45.9 109.5,45.6 v112.5,45.6
EXPANSIONB11  (via drill 0.3)
  Top 0.254: JP7.22 116.1,81 114.9,79.8 114.9,53.4 v115.2,53.1 116.4,51.9 116.4,51.3 JP5.22 116.4,51 116.4,50.7 114.9,49.2 114.9,48.3 115.8,47.4 115.8,26.1 115.5,25.8 115.5,25.2 115.8,24.9 115.8,22.5 116.1,22.2 116.1,21.3 JP9.22
  Bottom 0.254: v115.2,53.1 95.4,53.1 95.1,52.8 94.5,52.8 94.2,53.1 46.2,53.1 45.6,52.5 43.5,52.5 42.3,53.7 29.4,53.7 VENATRIX.26
EXPANSIONB12  (via drill 0.3)
  Top 0.254: JP9.24 118.8,21.3 118.8,22.2 117.6,23.4 117.6,49.2 118.8,50.4 118.8,51 JP5.24 118.8,51.3 118.8,52.2 117.6,53.4 v117.6,63.6 117.6,79.2 118.8,80.4 118.8,81 JP7.24
  Bottom 0.254: v117.6,63.6 54.6,63.6 48.3,69.9 25.2,69.9 24.6,69 24.6,57 25.5,56.1 28.2,56.1 VENATRIX.25
EXPANSIONB13  (via drill 0.3)
  Top 0.254: JP9.26 121.5,21.3 121.5,21.9 120,23.4 120,49.2 120.6,49.8 120.6,50.4 121.2,51 JP5.26 121.5,51.3 121.5,51.9 120,53.4 v120,62.4 120,79.8 121.2,81 JP7.26
  Bottom 0.254: v120,62.4 54.6,62.4 47.7,69.3 25.8,69.3 25.2,68.4 25.2,59.7 26.1,58.8 29.4,58.8 VENATRIX.24
EXPANSIONB14  (via drill 0.3)
  Top 0.254: JP9.28 123.9,21.3 123.9,22.2 122.7,23.4 122.7,49.2 123.3,49.8 123.3,50.7 123.6,51 JP5.28 123.9,51.3 123.9,52.2 122.7,53.4 v122.7,61.2 122.7,80.1 123.6,81 JP7.28
  Bottom 0.254: v122.7,61.2 54.6,61.2 47.1,68.7 26.4,68.7 25.8,67.8 25.8,61.8 26.4,61.2 29.4,61.2 VENATRIX.23
EXPANSIONB15  (via drill 0.3)
  Top 0.254: JP9.30 126.3,21.3 126.3,22.2 125.1,23.4 125.1,49.2 126.3,50.4 126.3,51 JP5.30 126.3,51.3 126.3,52.2 125.1,53.4 v125.1,60 125.1,79.2 126.3,80.4 126.3,81 JP7.30
  Bottom 0.254: v125.1,60 54.6,60 46.5,68.1 27,68.1 26.4,67.2 26.4,64.5 27.3,63.9 VENATRIX.22
EXPANSIONB16  (via drill 0.3)
  Top 0.254: JP9.32 129,21.3 129,21.9 127.8,23.1 127.8,49.2 128.4,49.8 128.4,50.7 JP5.32 129,51.3 129,51.9 127.8,53.1 v127.8,59.1 127.8,80.1 JP7.32
  Bottom 0.254: v127.8,59.1 54.3,59.1 45.9,67.5 32.1,67.5 31.2,66.3 29.4,66.3 VENATRIX.21
EXPANSIONB17  (via drill 0.3)
  Top 0.254: v54,1.8 54,4.8 52.8,6 52.8,6.9 JP4.34 | JP7.34 131.4,81 131.4,80.4 130.2,79.2 130.2,78.3 131.4,77.1 131.4,51.3 JP5.34 131.4,51 131.4,50.4 130.2,49.2 130.2,48.3 131.4,47.1 131.4,21.3 JP9.34 131.4,21 131.4,20.4 130.2,19.2 130.2,18.3 125.7,13.8 123.6,13.8 123,14.4 123,16.8 v122.7,17.1 | v64.8,18.9 64.8,4.5 JP2.1
  Bottom 0.254: v54,1.8 54.3,1.5 62.1,1.5 64.3,3.6 JP2.1 | v64.8,18.9 65.1,18.6 89.1,18.6 90.6,20.1 93.6,20.1 94.8,18.9 94.8,18.3 96.3,16.8 122.4,16.8 v122.7,17.1
EXPANSIONB18  (via drill 0.3)
  Top 0.254: JP7.36 134.1,81 134.1,80.7 135.3,79.5 135.3,78 134.1,76.8 v134.1,59.1 134.1,51.3 JP5.36 | v143.7,21.9 143.4,22.2 143.4,45.5 144.3,46.2 144.3,56.4 v141.9,58.8 | v67.8,6.3 70.1,4 JP2.2 | v53.1,31.8 56.1,28.8 56.1,13.8 55.2,12.9 55.2,7.2 JP4.36 | v133.5,30.6 133.2,30.3 133.2,24.9 134.1,24 134.1,21.3 JP9.36
  Bottom 0.254: v143.7,21.9 140.1,21.9 139.5,22.5 139.2,22.5 138.6,23.1 137.1,23.1 136.5,22.5 136.2,22.5 135,21.3 134.1,21.3 JP9.36 | v141.9,58.8 134.4,58.8 v134.1,59.1 | v67.8,6.3 65.1,9 59.4,9 58.5,8.1 57.3,8.1 56.1,6.9 55.5,6.9 JP4.36 | v53.1,31.8 53.4,31.8 53.7,32.1 105.3,32.1 105.6,31.8 127.2,31.8 128.4,30.6 v133.5,30.6
EXPANSIONB19  (via drill 0.3)
  Top 0.254: v137.1,56.4 136.5,55.8 136.5,51.3 JP5.38 136.5,51 136.5,50.4 135.3,49.2 135.3,48 136.5,46.8 136.5,21.3 JP9.38 | v140.1,56.4 139.8,56.7 139.8,76.5 141,77.7 v141,79.8 | v21.3,16.5 21,16.5 18,19.5 18,22.2 14.7,25.5 14.7,30.9 13.8,31.8 13.8,37.5 10.8,40.5 JP1.4 | v45.6,15.9 45.9,15.6 45.9,10.8 v45.6,10.5 | v57.9,9 57.9,7.2 JP4.38 | v90,17.4 87.3,14.7 v87,14.7
  Bottom 0.254: v140.1,56.4 v137.1,56.4 | v141,79.8 140.1,79.8 139.8,80.1 138.6,80.1 137.7,81 136.8,81 JP7.38 | v21.3,16.5 21.6,16.2 36.3,16.2 37.5,17.4 41.7,17.4 43.2,15.9 v45.6,15.9 | v45.6,10.5 46.2,9.9 57,9.9 57.3,9.6 | v57.9,9 57.3,9.6 | 68.2,9.6 72.6,3.7 JP2.3 68.2,9.6 | 57.3,9.6 68.2,9.6 | v90,17.4 93.6,17.4 94.8,16.2 123,16.2 125.1,18.3 125.1,19.2 126,20.1 134.7,20.1 135.3,20.7 136.2,20.7 136.5,21 JP9.38 | v87,14.7 86.7,15 68.2,15 68.2,9.6
EXPANSIONB20  (via drill 0.3, 0.6)
  Top 0.254: JP7.40 139.2,81 139.2,80.4 140.4,79.2 140.4,78 139.2,76.8 139.2,51.3 JP5.40 139.2,51 139.2,50.4 140.4,49.2 140.4,48 139.2,46.8 139.2,29.1 | 139.2,29.1 139.2,21.3 JP9.40 | v15.3,37.8 13.2,39.9 13.2,40.5 JP1.2 | v24.6,37.8 27.3,35.1 v27.3,24.3 | v35.1,24 35.1,18.3 v34.8,18 | v49.2,15.3 49.5,15 49.5,13.2 v51.9,10.8 | v60.3,10.5 60.3,7.2 JP4.40 60.3,6.9 60.3,6.6 62.4,4.5 62.4,3.6 v64.2,1.8 | v137.4,29.1 139.2,29.1 | v78.5,13.7 78.4,13.8 v78.4,30.6
  Bottom 0.254: v24.6,37.8 v15.3,37.8 | v27.3,24.3 30.3,24.3 30.9,23.7 34.8,23.7 v35.1,24 | v34.8,18 42,18 43.2,16.8 45.9,16.8 47.4,15.3 v49.2,15.3 | v51.9,10.8 52.2,10.5 v60.3,10.5 | v64.2,1.8 64.5,1.5 75.2,1.5 JP2.4 75.2,5.7 78.5,5.7 v78.5,13.7 | v137.4,29.1 118.2,29.1 116.7,30.6 105,30.6 104.7,30.9 78.5,30.9 v78.4,30.6
N$1
  Bottom 0.635: 41.1,93.9 38.7,93.9 VIN.2 | 41.1,93.9 45,93.9 D1.A | 41.1,93.9 41.1,90 40.2,89.1 39.6,89.1 38.7,88.2 38.7,86.4 VIN1.2
N$2  (via drill 0.61)
  Top 0.635: v50.1,81.8 v50.1,76.5 | v53.1,96 53.1,95.7 52.8,95.4 52.8,93.9 D1.C
  Bottom 0.635: v50.1,76.5 45.9,76.5 45.9,76.2 C1.+ | v50.1,81.8 50.1,82.4 51.9,82.4 53.1,83.7 53.1,93 52.5,93.6 52.5,93.9 52.8,93.9 D1.C | v53.1,96 53.7,96.6 62.4,96.6 IC3.1
N$3
  Bottom 0.254: D2.C 11.4,22.8 21.3,22.8 21.6,23.1 22.8,23.1 23.4,23.7 23.4,24.6 24.3,25.5 24.9,25.5 27,27.6 27.3,27.6 27.9,28.2 29.1,28.2 VENATRIX.36
N$4
  Bottom 0.254: VENATRIX.39 29.1,20.7 24,20.7 SW1.4
N$5
  Bottom 0.254: POWER.A 50.4,87 50.1,87.3 49.5,87.3 49.2,87 47.7,87 47.4,87.3 46.5,87.3 46.2,87 45.9,87 R1.2
N$6
  Bottom 0.254: VENATRIX.40 29.1,18 24,18 SW1.3
N$7  (via drill 0.3)
  Top 0.254: v41.7,35.7 42.3,35.7 43.5,36.9 45.9,36.9 46.5,36.3 46.5,34.8 47.1,34.2 47.1,8.1 46.2,7.2 46.2,6.3 45,5.1 45,4.5 JP4.27
  Bottom 0.254: v41.7,35.7 29.4,35.7 VENATRIX.33
N$65
  Bottom 0.254: Q3.2 23.3,40.8 29.1,40.8 VENATRIX.31
N$66
  Bottom 0.254: Q3.1 23.4,46.3 24.3,46.2 27,43.5 29.1,43.5 VENATRIX.30
VCC  (via drill 0.61)
  Top 0.635: 142.5,40.5 142.5,18.6 139.8,15.9 138.3,15.9 138,16.2 134.1,16.2 131.7,18.6 JP9.33 | v141.6,41.4 142.5,40.5 | v132.6,41.4 132.3,41.7 132.3,47.4 131.4,48.3 131.4,48.6 JP5.33 | 132.3,76.5 132.3,54.3 v132.9,53.7 | 132.3,76.5 132.3,77.4 131.7,78 131.7,78.6 JP7.33 | v142.8,53.7 142.5,53.4 142.5,40.5 | 61.5,80.1 61.5,88.2 67.8,94.5 67.8,96.6 IC3.3 | 61.5,80.1 61.5,78 D4.C | v48.6,79.8 45.9,82.5 45.9,84.3 R1.1 45.6,84.6 44.4,84.6 40.5,88.5 36.6,88.5 33,92.1 30.9,92.1 C30.1 30.6,92.1 v26.1,87.6 | v61.2,80.1 61.5,80.1 | v132.6,76.5 132.3,76.5 | IC4.1 16.5,96.6 15.6,95.7 15.6,92.7 C20.1 15.6,92.4 15.6,90.3 16.8,89.1 16.8,87.3 | 16.8,87.3 16.8,80.4 C2.+ | v17.1,87.3 16.8,87.3
  Bottom 0.635: v132.6,41.4 v141.6,41.4 | v142.8,53.7 v132.9,53.7 | v48.6,79.8 60.3,79.8 60.6,80.1 v61.2,80.1 73.8,80.1 77.4,76.5 v132.6,76.5 | v26.1,87.6 25.8,87.3 v17.1,87.3
VDD  (via drill 0.61)
  Top 0.635: v42.3,45.9 41.4,46.8 37.5,46.8 C29.1 37.2,46.8 33.2,46.8 | v33.2,38.7 33.2,46.8 | 22.5,26.7 22.5,26.4 | 24.6,24.3 R2.2 24.9,24.6 22.8,26.7 22.5,26.7 | 22.5,26.7 R3.1 22.2,26.7 22.2,29.1 21.9,29.4 21.9,30.6 R68.1 21.9,30.9 21.9,32.4 21.6,32.7 v21.6,33 21.9,33 23.4,34.5 23.4,38.1 24.3,39 27.3,39 27.9,38.4 29.1,38.4 VENATRIX.32 | v61.5,51.9 61.5,74.4 D5.C | v46.8,51.6 46.8,48 45.3,46.5 44.7,46.5 44.7,46.2 VENATRIX.12 | v137.7,46.5 137.4,46.8 137.4,47.1 136.5,48 136.5,48.6 JP5.37 | JP9.37 136.8,18.6 138,17.4 138.3,17.4 138.6,17.1 139.5,17.1 141.3,18.9 141.3,23.1 140.1,24.3 140.1,46.2 v140.4,46.5 141,46.5 141.3,46.8 141.3,56.7 140.7,57.3 140.7,75.6 v141,75.9 | v138,75.9 136.5,77.4 136.5,78.6 JP7.37 | v87.3,50.4 87.3,45 v88.5,43.8 | v133.8,43.5 133.5,43.8 133.5,46.5 134.1,47.1 134.1,48.6 JP5.35 | IC4.3 21.6,96.6 21.6,90 29.1,82.5 29.1,80.4 C3.+ 29.1,80.1 29.1,78 31.5,75.6 31.5,48.3 33,46.8 33.2,46.8
  Bottom 0.635: JP7.35 134.1,78.9 134.4,79.2 135.6,79.2 136.2,78.6 136.5,78.6 JP7.37 | JP9.35 134.1,18.9 134.4,19.2 135.6,19.2 136.2,18.6 136.5,18.6 JP9.37 | JP5.35 134.1,48.9 134.4,49.2 135.6,49.2 136.2,48.6 136.5,48.6 JP5.37 | v42.3,45.9 44.4,45.9 VENATRIX.12 | v33.2,38.7 31.2,38.7 30.9,38.4 29.7,38.4 VENATRIX.32 | v46.8,51.6 47.4,52.2 61.2,52.2 v61.5,51.9 61.5,51.6 63,50.1 87,50.1 v87.3,50.4 | v137.7,46.5 v140.4,46.5 | v141,75.9 v138,75.9 | v88.5,43.8 88.8,43.5 v133.8,43.5 | v21.6,33 19.8,33 17.7,35.1 16.5,35.1 IC2.8
VSS
  pour Bottom: 0.9,99.6 158.7,99.6 158.7,0.9 1.2,0.9 1.2,99.3
  pour Top: 1.2,99.9 158.7,99.9 158.7,1.2 1.2,1.2 1.2,99.3
(copper drawn outside any net)
  shapes: Bottom circle x8, Top circle x8

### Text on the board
Bottom: HIVE-BUS-Expansion | Zille9-2013
tPlace: 1
Measures: Modulbreite Anschlüsse rechts
Document: Variante mit 40-pol.Buchsenleiste, Module wahlweise senkrecht oder waagerecht (Ausrichtung nach rechts)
